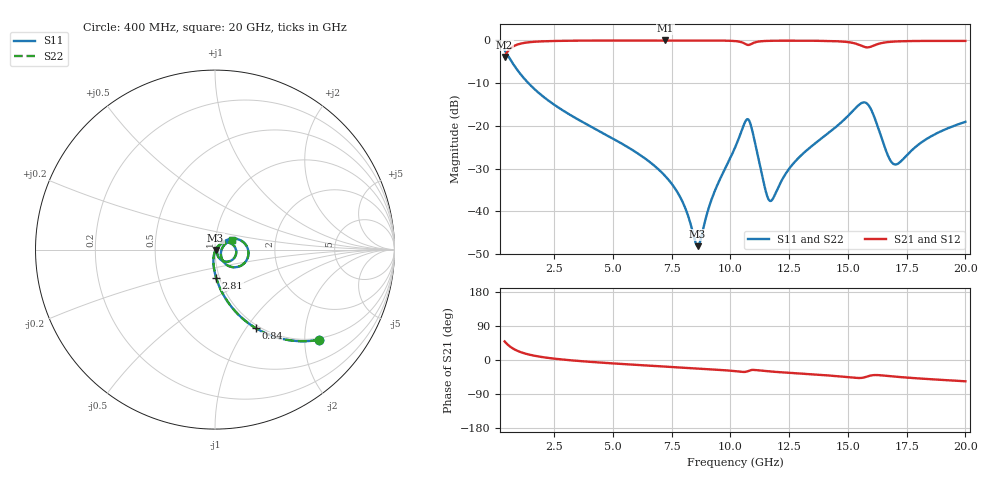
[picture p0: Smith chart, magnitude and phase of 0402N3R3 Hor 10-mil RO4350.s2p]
# MHz S  dB  R 50
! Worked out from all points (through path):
!   1961 points, 400 MHz to 20 GHz, reference 50 ohm
!   highest |S21| = -0.03 dB at 7.24 GHz (marker M1); lowest = -3.9 dB at 400 MHz (marker M2)
!   group delay of S21, straight-line fit = 10.1 ps
!   lowest |S11| = -48.1 dB at 8.61 GHz (marker M3), VSWR 1.01, Z = 50.4 - j0.178 ohm
!   |S11| at or under -10 dB: 1.41 GHz to end of sweep
!   |S22| runs from -48.1 to -2.3 dB; largest |S21 - S12| = 0
!   S11 on the Smith chart (normalised r, x): 400 MHz: 0.96, -2.34; 840 MHz: 0.96, -1.11; 2.81 GHz: 0.96, -0.31; 20 GHz: 1.21, +0.13
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400  -2.30 -40.9  -3.86 49.1  -3.86 49.1  -2.30 -40.9
840  -6.14 -62.6  -1.22 27.3  -1.22 27.3  -6.14 -62.6
1510  -10.56 -76.5  -0.41 13.3  -0.41 13.3  -10.56 -76.5
2810  -16.15 -87.8  -0.12 1.6  -0.12 1.6  -16.15 -87.8
3670  -18.96 -92.2  -0.07 -3.1  -0.07 -3.1  -18.96 -92.2
6940  -30.15 -101.0  -0.03 -16.3  -0.03 -16.3  -30.15 -101.0
7240  -31.79 -100.7  -0.03 -17.4  -0.03 -17.4  -31.79 -100.7
7960  -37.66 -95.2  -0.03 -20.0  -0.03 -20.0  -37.66 -95.2
8610  -48.14 -26.9  -0.04 -22.3  -0.04 -22.3  -48.14 -26.9
9280  -36.07 45.6  -0.05 -24.9  -0.05 -24.9  -36.07 45.6
10200  -25.10 41.5  -0.18 -29.4  -0.18 -29.4  -25.10 41.5
10790  -18.67 -24.1  -1.08 -28.3  -1.08 -28.3  -18.67 -24.1
11510  -35.31 -47.3  -0.15 -29.3  -0.15 -29.3  -35.31 -47.3
11710  -37.57 -11.8  -0.11 -30.4  -0.11 -30.4  -37.57 -11.8
12530  -29.83 41.2  -0.08 -33.9  -0.08 -33.9  -29.83 41.2
13470  -24.71 43.1  -0.10 -37.7  -0.10 -37.7  -24.71 43.1
15710  -14.51 -12.4  -1.55 -45.8  -1.55 -45.8  -14.51 -12.4
16040  -16.79 -42.8  -1.36 -40.3  -1.36 -40.3  -16.79 -42.8
16740  -27.36 -40.1  -0.39 -42.4  -0.39 -42.4  -27.36 -40.1
17110  -28.91 -4.8  -0.25 -44.5  -0.25 -44.5  -28.91 -4.8
18370  -23.00 29.4  -0.14 -50.1  -0.14 -50.1  -23.00 29.4
20000  -19.06 29.1  -0.14 -56.2  -0.14 -56.2  -19.06 29.1
